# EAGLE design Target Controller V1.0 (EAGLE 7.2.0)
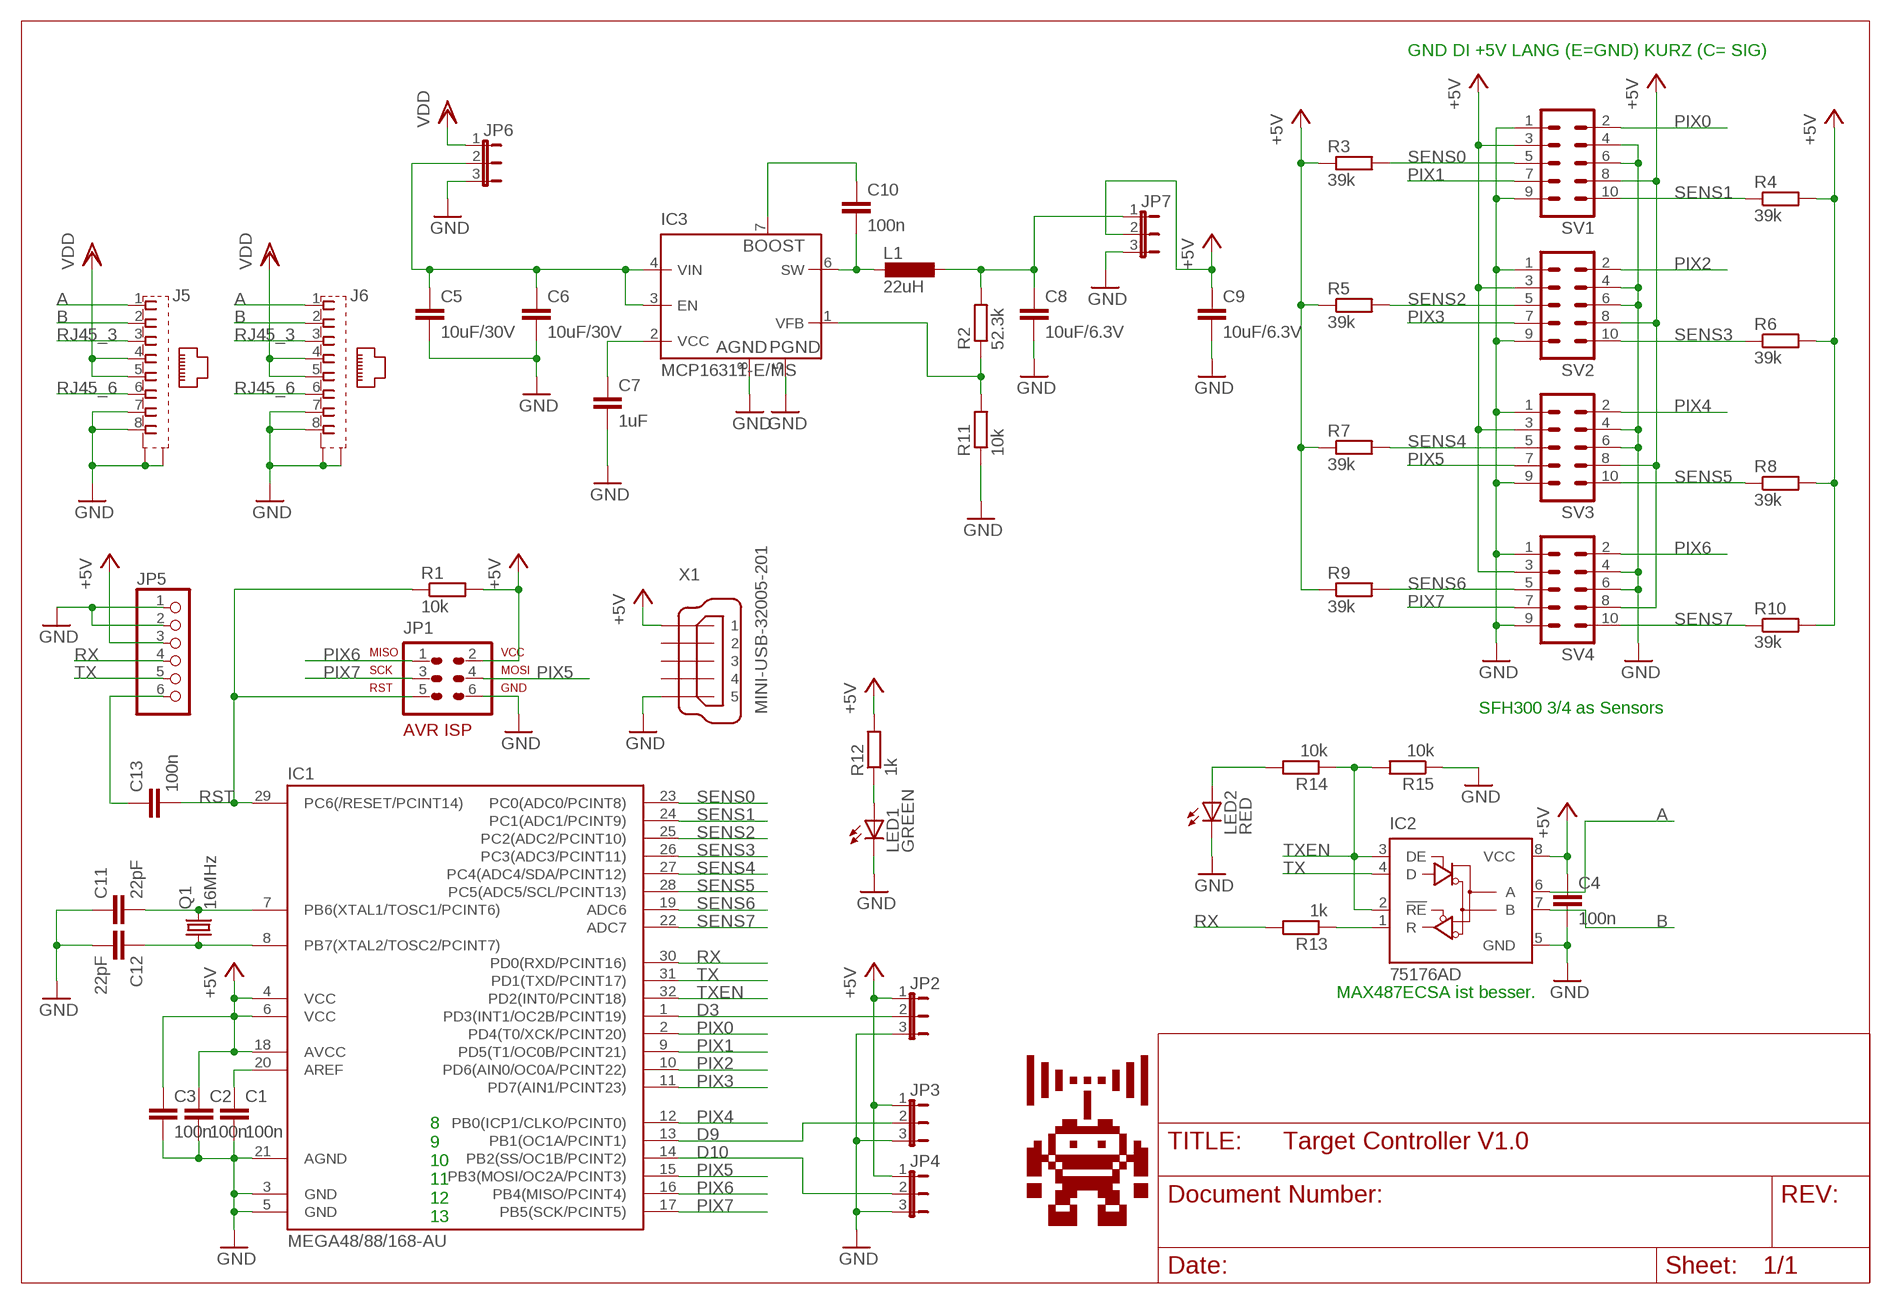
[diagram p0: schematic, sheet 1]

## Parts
C1  100n  C-EUC0805K  [C0805K]
C2  100n  C-EUC0805K  [C0805K]
C3  100n  C-EUC0805K  [C0805K]
C4  100n  C-EUC0805K  [C0805K]
C5  10uF/30V  C-EUC1206K  [C1206K]
C6  10uF/30V  C-EUC1206K  [C1206K]
C7  1uF  C-EUC0805K  [C0805K]
C8  10uF/6.3V  C-EUC0805K  [C0805K]
C9  10uF/6.3V  C-EUC0805K  [C0805K]
C10  100n  C-EUC0805K  [C0805K]
C11  22pF  C-EUC0603K  [C0603K]
C12  22pF  C-EUC0603K  [C0603K]
C13  100n  C-EUC0805K  [C0805K]
IC1  MEGA48/88/168-AU  [TQFP32-08]
IC2  75176AD  [D_R-PDSO-G8]
IC3  MCP16311-E/MS  MCP16311  [MSOP8]
J5  MEBP8-8G  [MEBP8-8G]
J6  MEBP8-8G  [MEBP8-8G]
JP1  AVR-ISP-6VERT  [AVR-ISP-6]
JP2  JP2E  [JP2]
JP3  JP2E  [JP2]
JP4  JP2E  [JP2]
JP5  PINHD-1X6  [1X06]
JP6  JP2E  [JP2]
JP7  JP2E  [JP2]
L1  22uH  L-PISM  [L-PISM22]
LED1  GREEN  LEDCHIPLED_0805  [CHIPLED_0805]
LED2  RED  LEDCHIPLED_0805  [CHIPLED_0805]
Q1  16MHz  CRYSTALHC49UP  [HC49UP]
R1  10k  R-EU_R0805  [R0805]
R2  52.3k  R-EU_R0805  [R0805]
R3  39k  R-EU_R0805  [R0805]
R4  39k  R-EU_R0805  [R0805]
R5  39k  R-EU_R0805  [R0805]
R6  39k  R-EU_R0805  [R0805]
R7  39k  R-EU_R0805  [R0805]
R8  39k  R-EU_R0805  [R0805]
R9  39k  R-EU_R0805  [R0805]
R10  39k  R-EU_R0805  [R0805]
R11  10k  R-EU_R0805  [R0805]
R12  1k  R-EU_R0805  [R0805]
R13  1k  R-EU_R0805  [R0805]
R14  10k  R-EU_R0805  [R0805]
R15  10k  R-EU_R0805  [R0805]
SV1  ML10L  [ML10L]
SV2  ML10L  [ML10L]
SV3  ML10L  [ML10L]
SV4  ML10L  [ML10L]
U$1  HACKFFM_LOGOLOGO_BSTOP  [LOGO_BSTOP]
X1  MINI-USB-32005-201  [32005-201]

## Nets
+5V: C2.1 C3.1 C4.1 C9.1 IC1.4(VCC) IC1.6(VCC) IC1.18(AVCC) IC2.8(VCC) JP1.2 JP2.1 JP3.1 JP4.1 JP5.3 JP7.2 R1.2 R3.1 R4.2 R5.1 R6.2 R7.1 R8.2 R9.1 R10.2 R12.2 SV1.3 SV1.8 SV2.3 SV2.8 SV3.3 SV3.8 SV4.3 SV4.8 X1.1
A: IC2.6(A) J5.1 J6.1
AREF: C1.1 IC1.20(AREF)
B: IC2.7(B) J5.2 J6.2
D3: IC1.1(PD3(INT1/OC2B/PCINT19)) JP2.2
D9: IC1.13(PB1(OC1A/PCINT1)) JP3.2
D10: IC1.14(PB2(SS/OC1B/PCINT2)) JP4.2
GND: C1.2 C2.2 C3.2 C4.2 C5.2 C6.2 C7.2 C8.2 C9.2 C11.1 C12.2 IC1.3(GND) IC1.5(GND) IC1.21(AGND) IC2.5(GND) IC3.5(PGND) IC3.8(AGND) J5.7 J5.8 J5.S1 J5.S2 J6.7 J6.8 J6.S1 J6.S2 JP1.6 JP2.3 JP3.3 JP4.3 JP5.1 JP5.2 JP6.3 JP7.3 LED1.C LED2.C R11.1 R15.1 SV1.1 SV1.4 SV1.6 SV1.9 SV2.1 SV2.4 SV2.6 SV2.9 SV3.1 SV3.4 SV3.6 SV3.9 SV4.1 SV4.4 SV4.6 SV4.9 X1.5
N$8: C10.1 IC3.7(BOOST)
N$9: C7.1 IC3.2(VCC)
N$11: C8.1 JP7.1 L1.2 R2.2
N$12: C12.1 IC1.8(PB7(XTAL2/TOSC2/PCINT7)) Q1.1
N$13: C11.2 IC1.7(PB6(XTAL1/TOSC1/PCINT6)) Q1.2
N$14: IC2.1(R) R13.1
N$15: LED1.A R12.1
N$16: C13.1 JP5.6
N$17: LED2.A R14.2
PIX0: IC1.2(PD4(T0/XCK/PCINT20)) SV1.2
PIX1: IC1.9(PD5(T1/OC0B/PCINT21)) SV1.7
PIX2: IC1.10(PD6(AIN0/OC0A/PCINT22)) SV2.2
PIX3: IC1.11(PD7(AIN1/PCINT23)) SV2.7
PIX4: IC1.12(PB0(ICP1/CLKO/PCINT0)) SV3.2
PIX5: IC1.15(PB3(MOSI/OC2A/PCINT3)) JP1.4 SV3.7
PIX6: IC1.16(PB4(MISO/PCINT4)) JP1.1 SV4.2
PIX7: IC1.17(PB5(SCK/PCINT5)) JP1.3 SV4.7
RJ45_3: J5.3 J6.3
RJ45_6: J5.6 J6.6
RST: C13.2 IC1.29(PC6(/RESET/PCINT14)) JP1.5 R1.1
RX: IC1.30(PD0(RXD/PCINT16)) JP5.4 R13.2
SENS0: IC1.23(PC0(ADC0/PCINT8)) R3.2 SV1.5
SENS1: IC1.24(PC1(ADC1/PCINT9)) R4.1 SV1.10
SENS2: IC1.25(PC2(ADC2/PCINT10)) R5.2 SV2.5
SENS3: IC1.26(PC3(ADC3/PCINT11)) R6.1 SV2.10
SENS4: IC1.27(PC4(ADC4/SDA/PCINT12)) R7.2 SV3.5
SENS5: IC1.28(PC5(ADC5/SCL/PCINT13)) R8.1 SV3.10
SENS6: IC1.19(ADC6) R9.2 SV4.5
SENS7: IC1.22(ADC7) R10.1 SV4.10
SW: C10.2 IC3.6(SW) L1.1
TX: IC1.31(PD1(TXD/PCINT17)) IC2.4(D) JP5.5
TXEN: IC1.32(PD2(INT0/PCINT18)) IC2.2(!RE) IC2.3(DE) R14.1 R15.2
VDD: J5.4 J5.5 J6.4 J6.5 JP6.1
VFB: IC3.1(VFB) R2.1 R11.2
VIN: C5.1 C6.1 IC3.3(EN) IC3.4(VIN) JP6.2
Unconnected: X1.2 X1.3 X1.4

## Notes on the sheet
- GND DI +5V LANG (E=GND) KURZ (C= SIG)
- SFH300 3/4 as Sensors
- MAX487ECSA ist besser.
- 8
  9
  10
  11
  12
  13

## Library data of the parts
C1-C13 = rcl:C-EU: CAPACITOR, European symbol
IC1 = avr-7:MEGA48/88/168
IC2 = 751xx:75176A: DIFFERENTIAL BUS TRANSCEIVER Source: http://focus.ti.com/lit/ds/symlink/sn75176a.pdf
IC3 = Lutz:MCP16311
J5 J6 = Lutz:MEBP8-8G
JP1 = avr-7:AVR-ISP-6: AVR ISP-6 Serial Programming Header
JP2-JP4 JP6 JP7 = jumper:JP2E: JUMPER
JP5 = pinhead:PINHD-1X6: PIN HEADER
L1 = Lutz:L-PISM
LED1 LED2 = led:LED: LED
Q1 = crystal:CRYSTAL: CRYSTAL; OC_FARNELL: unknown; OC_NEWARK: unknown
R1-R15 = rcl:R-EU_: RESISTOR, European symbol
SV1-SV4 = con-ml:ML10L: HARTING; OC_FARNELL: unknown; OC_NEWARK: unknown
U$1 = hackffm_logo:HACKFFM_LOGO
X1 = con-cypressindustries:MINI-USB-: MINI USB-B Conector Source: www.cypressindustries.com; OC_FARNELL: unknown; OC_NEWARK: unknown

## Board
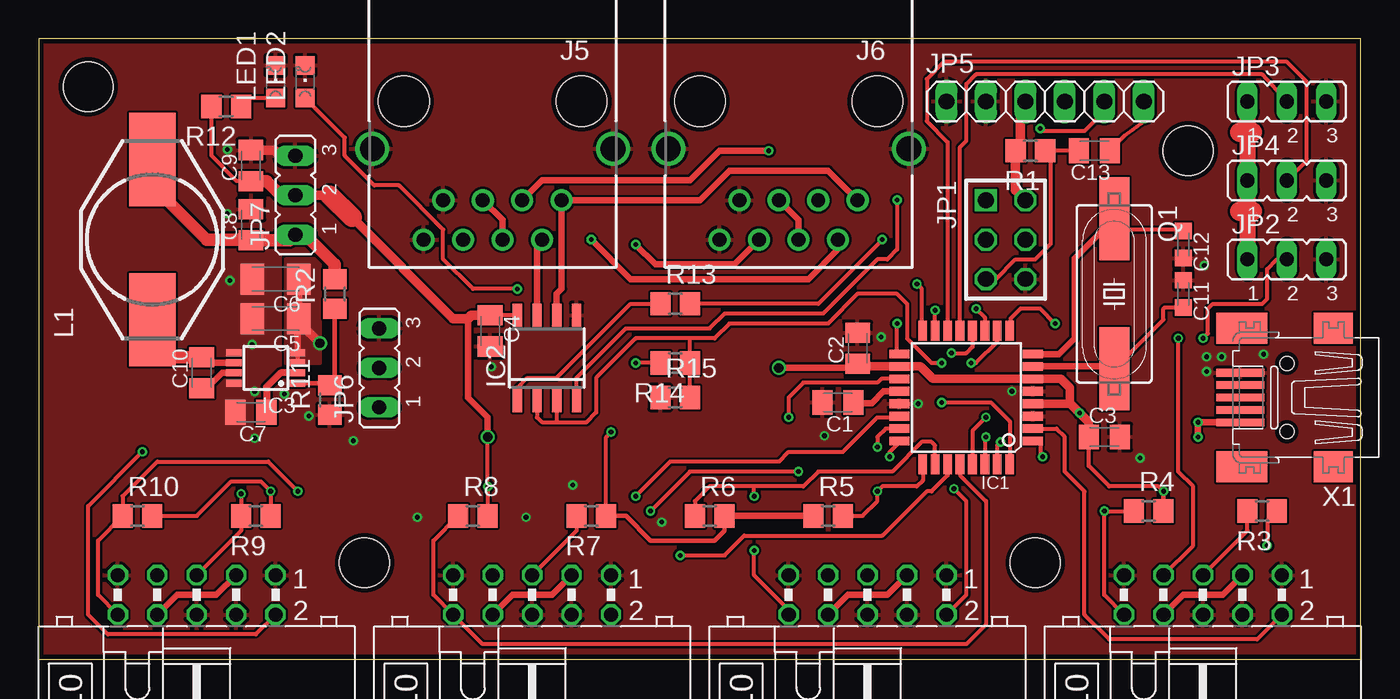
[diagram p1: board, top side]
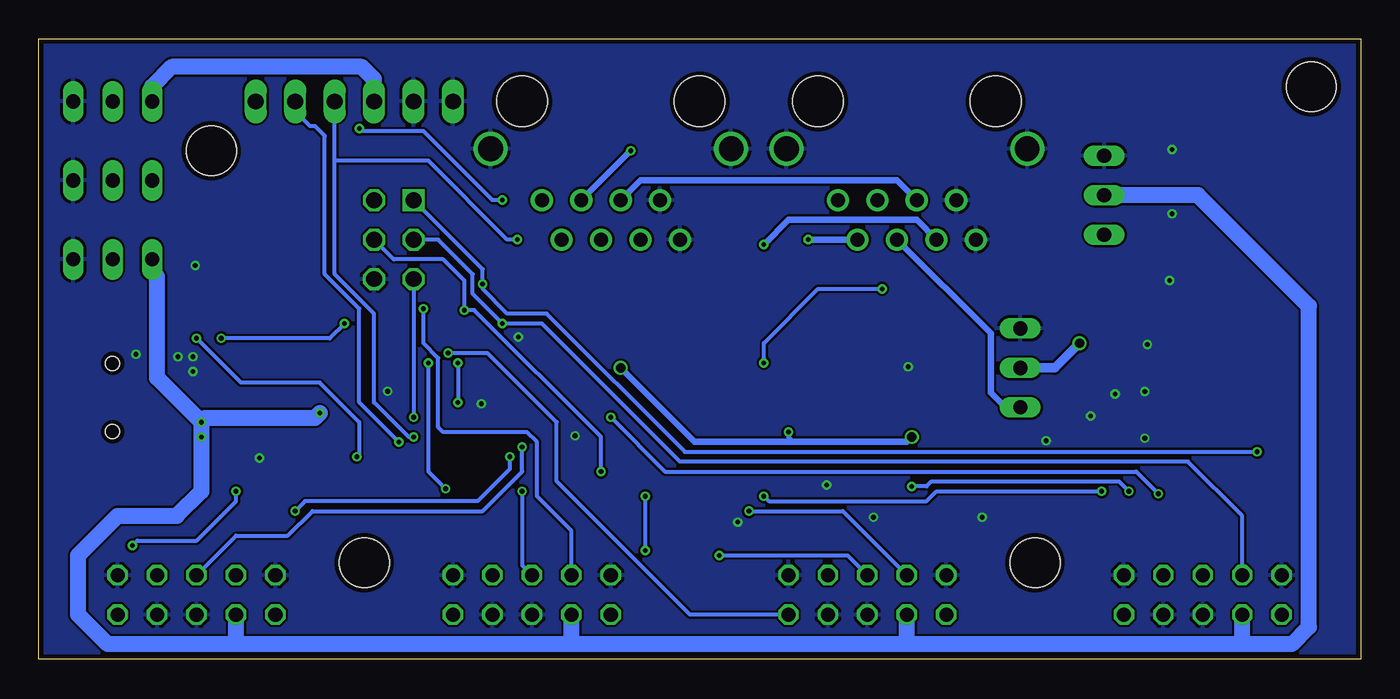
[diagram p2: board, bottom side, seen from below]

Size 85.08 x 39.91 mm. Coordinates in mm from the lower left corner, seen from the top.
Outline: 0,0 85.08,0 85.08,39.91 0,39.91 0,0
Copper layers (1*16): Top 0.035mm / dielectric 1.5mm / Bottom 0.035mm
Design rules "PCB-POOL Standard *": minimum track width 0.15mm, minimum drill 0.3mm, track to track 0.15mm, track to pad 0.15mm, pad to pad 0.15mm, via to via 0.15mm, smd to smd 0.15mm, copper to edge 0.3mm, drill to drill 0.2mm, minimum pad ring 0.2mm, minimum via ring 0.15mm, stop-mask expansion 0.075mm, vias tented up to drill 0.3mm, thermal gap 0.2mm
Holes 3.2 mm at 3.17,36.83 73.98,32.7 64.14,6.19 20.95,6.19

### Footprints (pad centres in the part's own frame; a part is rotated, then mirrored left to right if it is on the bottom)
C0805K = smd 1.3 x 1.6: 1 -1,0; 2 1,0
C1206K = smd 1.5 x 2: 1 -1.5,0; 2 1.5,0
C0603K = smd 1.05 x 1.08: 1 -0.875,0; 2 0.875,0
TQFP32-08 = smd 1.27 x 0.559: 1 -4.293,2.8; 2 -4.293,2; 3 -4.293,1.2; 4 -4.293,0.4; 5 -4.293,-0.4; 6 -4.293,-1.2; 7 -4.293,-2; 8 -4.293,-2.8; 17 4.293,-2.8; 18 4.293,-2; 19 4.293,-1.2; 20 4.293,-0.4; 21 4.293,0.4; 22 4.293,1.2; 23 4.293,2; 24 4.293,2.8 | smd 0.559 x 1.27: 9 -2.8,-4.293; 10 -2,-4.293; 11 -1.2,-4.293; 12 -0.4,-4.293; 13 0.4,-4.293; 14 1.2,-4.293; 15 2,-4.293; 16 2.8,-4.293; 25 2.8,4.293; 26 2,4.293; 27 1.2,4.293; 28 0.4,4.293; 29 -0.4,4.293; 30 -1.2,4.293; 31 -2,4.293; 32 -2.8,4.293
D_R-PDSO-G8 = smd 0.6 x 1.5: 1 -1.905,-2.75; 2 -0.635,-2.75; 3 0.635,-2.75; 4 1.905,-2.75; 5 1.905,2.75; 6 0.635,2.75; 7 -0.635,2.75; 8 -1.905,2.75
MSOP8 = smd 0.45 x 1: 1 -0.975,-2.05; 2 -0.325,-2.05; 3 0.325,-2.05; 4 0.975,-2.05; 5 0.975,2.05; 6 0.325,2.05; 7 -0.325,2.05; 8 -0.975,2.05
MEBP8-8G = drill 0.9 pad 1.422: 1 -4.445,-2.54; 2 -3.175,0; 3 -1.905,-2.54; 4 -0.635,0; 5 0.635,-2.54; 6 1.905,0; 7 3.175,-2.54; 8 4.445,0 | drill 1.6 pad 2.184: S1 -7.745,-5.84; S2 7.745,-5.84 | hole 3.25: 5.715,-8.89; -5.715,-8.89
AVR-ISP-6 = drill 1.016 square: 1 -2.54,-1.27 | drill 1.016 octagon: 2 -2.54,1.27; 3 0,-1.27; 4 0,1.27; 5 2.54,-1.27; 6 2.54,1.27
JP2 = drill 0.914 long: 1 -2.54,0; 2 0,0; 3 2.54,0
1X06 = drill 1.016 long: 1 -6.35,0; 2 -3.81,0; 3 -1.27,0; 4 1.27,0; 5 3.81,0; 6 6.35,0
L-PISM22 = smd 6 x 3: 1 -5.15,0; 2 5.15,0
CHIPLED_0805 = smd 1.2 x 1.2: A 0,-1.05; C 0,1.05
HC49UP = smd 5.334 x 1.93: 1 -4.826,0; 2 4.826,0
R0805 = smd 1.3 x 1.5: 1 -0.95,0; 2 0.95,0
ML10L = drill 0.914 octagon: 1 -5.08,-1.27; 2 -5.08,1.27; 3 -2.54,-1.27; 4 -2.54,1.27; 5 0,-1.27; 6 0,1.27; 7 2.54,-1.27; 8 2.54,1.27; 9 5.08,-1.27; 10 5.08,1.27
32005-201 = smd 3.1 x 0.5: 1 3,1.6; 2 3,0.8; 3 3,0; 4 3,-0.8; 5 3,-1.6 | smd 2.5 x 2: M1 -3,-4.45; M2 -3,4.45 | smd 3.3 x 2: M3 2.9,4.45; M4 2.9,-4.45 | hole 0.9: 0,2.2; 0,-2.2

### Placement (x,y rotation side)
C1  51.44,16.51 180 top
C2  52.7,20 90 top
C3  68.58,14.29 0 top
C4  29.05,21.11 270 top
C5  15.24,21.91 180 top
C6  15.24,24.45 180 top
C7  13.65,15.88 180 top
C8  13.65,27.94 90 top
C9  13.65,31.75 90 top
C10  10.48,18.41 90 top
C11  73.66,23.5 270 top
C12  73.66,26.67 270 top
C13  67.94,32.7 180 top
IC1  59.69,16.83 180 top
IC2  32.7,19.37 0 top
IC3  14.61,18.73 90 top
J5  29.21,26.99 180 top
J6  48.26,26.99 180 top
JP1  62.23,26.99 270 top
JP2  80.33,25.72 0 top
JP3  80.33,35.88 0 top
JP4  80.33,30.8 0 top
JP5  64.77,35.88 0 top
JP6  21.91,18.73 90 top
JP7  16.51,29.84 90 top
L1  7.3,26.99 90 top
LED1  15.24,37.15 0 top
LED2  17.14,37.15 0 top
Q1  69.22,23.5 270 top
R1  63.82,32.7 180 top
R2  19.05,23.5 90 top
R3  78.74,9.53 180 top
R4  71.44,9.53 0 top
R5  50.8,9.21 0 top
R6  43.18,9.21 0 top
R7  35.56,9.21 180 top
R8  27.94,9.21 0 top
R9  13.97,9.21 180 top
R10  6.35,9.21 0 top
R11  18.73,16.67 90 top
R12  12.06,35.56 180 top
R13  40.96,22.86 0 top
R14  40.96,19.05 180 top
R15  40.96,16.83 0 top
SV1  74.93,4.13 180 top
SV2  53.34,4.13 180 top
SV3  31.75,4.13 180 top
SV4  10.16,4.13 180 top
U$1  8.73,19.68 270 top
X1  80.33,16.83 180 top

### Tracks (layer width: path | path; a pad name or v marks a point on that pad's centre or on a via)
+5V  (via drill 0.3, 0.6)
  Top 0.254: 78.11,28.81 77.79,29.13 77.79,31.75 | 78.11,33.89 77.79,34.21 JP3.1 | v72.39,10.79 R4.2 v72.39,10.79 | v72.39,10.79 72.07,11.11 68.9,11.11 67.58,12.43 C3.1 | R3.1 79.06,8.89 v79.06,7.3 | IC2.8 C4.1 | C9.1 12.75,30.75 11.11,32.38 R12.2 | R10.2 10.16,9.21 12.38,11.43 14.29,11.43 v14.92,10.79 R9.1 | v28.89,14.29 v28.89,11.11 R8.2 | R7.1 36.51,14.29 v36.83,14.61
  Top 0.305: R7.1 37.78,9.21 39.37,7.62 43.5,7.62 44.13,8.26 R6.2
  Top 0.406: SV4.8 8.89,4.13 11.43,4.13 SV4.3 | SV3.8 30.48,4.13 33.02,4.13 SV3.3 | SV2.8 52.07,4.13 54.61,4.13 SV2.3 | SV1.8 73.66,4.13 76.2,4.13 SV1.3 | X1.1 77.31,15.24 v74.61,15.24 v74.61,14.29 | 49.53,8.89 R5.1 R6.2 | R10.2 | R9.1 | R8.2 | C2.1 52.44,19 | 52.44,18.73 v47.62,18.73 | 27.62,21.91 27.62,16.83 28.89,15.56 v28.89,14.29
  Top 0.559: C2.1 52.53,18.83 IC1.18 56.74,18.83 57.54,18.03 IC1.6 65.79,18.03 66.36,17.46 66.36,16.46 v66.99,15.83 | IC1.4 66.39,16.43 v66.99,15.83 | C3.1 67.58,15.24 v66.99,15.83
  Top 0.61: JP7.2 18.73,29.84 | JP5.3 63.18,35.56 63.18,33.02 R1.2 62.87,30.16 JP1.2 | 20.16,28.42 26.67,21.91 27.62,21.91 27.83,22.12 C4.1 | C2.1 52.44,18.73
  Top 0.813: C9.1 14.65,30.75 15.56,29.84 JP7.2
  Top 1.016: JP2.1 JP4.1 77.79,31.75 JP3.1
  Top 1.27: 18.73,29.84 20.16,28.42 | 77.31,33.89 78.11,33.89 | 77.31,28.81 78.11,28.81
  Bottom 0.254: v79.06,7.3 78.74,7.62 74.93,7.62 72.39,10.16 v72.39,10.79 | v14.92,10.79 15.56,11.43 27.62,11.43 27.94,11.11 v28.89,11.11 | v36.83,14.61 36.83,14.29 36.51,13.97
  Bottom 0.406: v28.89,14.29 29.21,13.97 36.51,13.97 42.86,13.97 v47.62,18.73
  Bottom 1.016: 7.62,0.95 4.45,0.95 3.33,2.06 3.33,22.7 10.48,29.84 JP7.2 | 7.62,0.95 29.21,0.95 | 29.21,0.95 50.8,0.95 | 50.8,0.95 72.39,0.95 | 72.39,0.95 80.64,0.95 82.55,2.86 82.55,6.67 80.01,9.21 76.2,9.21 74.61,10.79 v74.61,15.24 | 72.39,0.95 SV1.8 | 50.8,0.95 SV2.8 | 29.21,0.95 SV3.8 | 7.62,0.95 SV4.8 | v74.61,15.24 77.47,18.1 77.47,24.61 77.79,24.92 JP2.1 | v74.61,15.24 74.34,15.51 67.31,15.51 v66.99,15.83 | JP5.3 63.5,37.31 64.29,38.1 76.52,38.1 77.79,36.83 JP3.1
A
  Top 0.406: IC2.6 33.34,23.5 33.66,23.81 J5.1 42.55,29.53 44.45,31.43 50.8,31.43 J6.1
AREF
  Top 0.406: IC1.20 54.38,17.23 53.61,16.46 52.48,16.46 C1.1
B  (via drill 0.3)
  Top 0.406: J5.2 32.07,26.67 IC2.7 | v35.56,26.99 38.1,24.45 49.53,24.45 51.44,26.35 J6.2
  Bottom 0.406: J5.2 v35.56,26.99
D3  (via drill 0.3)
  Top 0.254: IC1.1 64.45,14.03 64.45,13.18 v64.61,13.02 | v74.93,20.64 75.25,20.95 75.25,22.54 75.56,22.86 78.74,22.86 79.06,23.18 79.06,25.08 79.69,25.72 JP2.2
  Bottom 0.254: v64.61,13.02 64.45,13.18 64.45,15.24 66.99,17.78 72.07,17.78 v74.93,20.64
D9
  Top 0.254: JP3.2 78.74,37.62 60.33,37.62 59.69,36.99 59.69,33.34 59.29,32.94 IC1.13
D10
  Top 0.254: JP4.2 81.6,32.07 81.6,37.15 80.33,38.42 58.26,38.42 57.15,37.31 57.15,34.61 58.49,33.27 IC1.14
GND  (via drill 0.3)
  Top 0.406: IC3.8 12.34,17.76
  Top 0.61: C9.2 15.19,32.75 15.56,32.38 JP7.3
  other vias: 56.6,16.43 62.63,17.23 13.73,20.24 13.89,17.22 17.39,15.63 13.89,14.21 15.8,17.06 12.15,32.78 12.15,28.65 12.31,24.36 31.36,9.12 24.37,9.12 40.09,8.81 34.37,11.19 20.24,14.05 29.13,18.81 78.82,19.61 76.12,19.45 70.89,12.94 54.22,20.72 75.01,25.32 75.17,19.45 75.17,18.5 50.56,14.36
  pour Bottom: 0,0 0,40.64 85.09,40.64 85.09,0
  pour Top (rank 2): 0,0 0,40.64 85.09,40.64 85.09,0
  pour Top (no thermals): 11.75,25.72 14.92,25.72 14.92,14.61 11.43,14.61 11.43,25.72
N$8
  Top 0.406: IC3.7 11.79,18.41 10.79,17.41 C10.1
N$9
  Top 0.457: IC3.2 15.55,18.41 14.65,17.51 C7.1
N$11
  Top 0.813: 7.62,31.43 L1.2 6.99,30.8 10.79,26.99 13.61,26.99 C8.1 16.14,26.94 JP7.1 17.14,27.3 19.05,25.4 R2.2
N$12
  Top 0.254: C12.1 73.58,27.62 69.22,27.62
  Top 0.406: 69.22,26.04 69.22,27.62 Q1.1 | 69.22,27.86 Q1.1 | IC1.8 65.67,19.63 66.67,20.64 66.67,25.78 Q1.1 | 69.39,28.18 Q1.1
N$13
  Top 0.254: Q1.2 72.39,21.84 72.39,22.54 72.47,22.62 C11.2
  Top 0.406: IC1.7 69.22,18.83 Q1.2 69.22,21.03
N$14
  Top 0.254: R13.1 38.1,22.86 33.34,18.1 31.43,18.1 30.8,17.46 IC2.1
N$15
  Top 0.254: LED1.A 13.55,36.1 R12.1
N$16
  Top 0.254: C13.1 69.9,33.7 71.12,34.61 JP5.6
N$17  (via drill 0.3)
  Top 0.254: R14.2 v38.42,19.05 | v30.8,23.81 27.94,23.81 26.04,25.72 26.04,27.62 23.18,30.48 21.59,30.48 19.68,32.38 19.68,33.56 LED2.A
  Bottom 0.254: v38.42,19.05 38.42,20.32 34.92,23.81 v30.8,23.81
PIX0
  Top 0.254: IC1.2 65.5,14.83 66.04,14.29 66.04,12.06 67.31,10.79 67.31,2.86 68.9,1.27 78.42,1.27 SV1.2
PIX1  (via drill 0.3)
  Top 0.254: 62.49,21.59 IC1.9 62.49,21.53 62.55,21.59 62.55,21.91 63.18,22.54 64.45,22.54 v65.41,21.59 | v73.34,20.64 73.34,12.06 74.3,11.11 74.3,7.3 SV1.7
  Bottom 0.254: v65.41,21.59 66.36,20.64 v73.34,20.64
PIX2  (via drill 0.3)
  Top 0.254: IC1.10 61.69,20.41 60.33,19.05 v60.01,19.05 | SV2.2 59.69,4.13 59.69,10.16 v58.9,10.95
  Bottom 0.254: v58.9,10.95 60.01,12.06 v60.01,19.05
PIX3  (via drill 0.3)
  Top 0.254: v60.33,22.54 60.89,21.98 IC1.11
  Bottom 0.254: SV2.7 50.8,8.26 53.02,10.48 53.02,13.97 53.66,14.61 59.05,14.61 59.37,14.92 59.37,19.37 60.33,20.32 v60.33,22.54
PIX4  (via drill 0.3)
  Top 0.254: IC1.12 60.09,20.09 59.69,19.68 v58.74,19.68
  Bottom 0.254: SV3.2 43.18,2.86 51.75,11.43 51.75,15.24 56.2,19.68 v58.74,19.68
PIX5  (via drill 0.3)
  Top 0.254: IC1.15 v57.69,22.45 | v48.9,12.06 41.91,12.06 v39.37,9.53
  Bottom 0.254: JP1.4 62.23,25.72 59.05,25.72 57.69,24.35 v57.69,22.45 57.05,22.45 48.9,14.29 v48.9,12.06 | v39.37,9.53 33.34,9.53 SV3.7
PIX6  (via drill 0.3)
  Top 0.254: SV4.2 13.97,1.59 4.45,1.59 3.17,2.86 3.17,9.84 v6.67,13.34 | 56.83,21.18 56.83,23.81 v56.52,24.13
  Top 0.406: 56.83,21.18 IC1.16
  Bottom 0.254: v6.67,13.34 43.5,13.34 52.39,22.23 54.93,22.23 56.52,23.81 v56.52,24.13 56.52,25.08 JP1.1
PIX7  (via drill 0.3)
  Top 0.254: IC1.17 55.24,19.63 v55.24,21.59
  Bottom 0.254: JP1.3 59.37,26.99 57.15,24.77 57.15,23.5 v55.24,21.59 52.7,21.59 43.81,12.7 11.11,12.7 7.62,9.21 SV4.7
RJ45_3  (via drill 0.3)
  Top 0.406: J5.3 32.38,30.8 41.91,30.8 43.81,32.7 v46.99,32.7
  Bottom 0.406: J6.3 v46.99,32.7
RJ45_6  (via drill 0.3)
  Top 0.406: v38.42,26.67 39.69,25.4 44.77,25.4 J6.6
  Bottom 0.406: J5.6 28.57,28.26 36.83,28.26 v38.42,26.67
RST  (via drill 0.3)
  Top 0.254: IC1.29 60.09,14.69 v60.96,15.56 | JP1.5 61.59,24.45 62.87,25.72 64.14,25.72 65.13,26.71 65.13,32.59 R1.1 C13.2
  Bottom 0.254: JP1.5 v60.96,15.56
RX  (via drill 0.3)
  Top 0.254: v60.96,14.29 60.89,14.22 IC1.30 | v54.29,26.99 50.16,22.86 R13.2
  Bottom 0.254: 66.04,32.07 66.04,24.77 63.5,22.23 63.5,16.51 61.28,14.29 v60.96,14.29 | 66.04,32.07 JP5.4 | v54.29,26.99 54.93,26.99 60.01,32.07 66.04,32.07
SENS0  (via drill 0.3)
  Top 0.254: SV1.5 77.79,8.26 R3.2 | IC1.23 54.52,14.83 53.98,14.29 v53.98,13.65
  Bottom 0.254: SV1.5 72.39,7.94 69.06,7.94 67.47,9.53 56.52,9.53 53.98,12.06 v53.98,13.65
SENS1  (via drill 0.3)
  Top 0.254: SV1.10 68.58,4.13 v68.58,9.53 R4.1 | IC1.24 55.46,14.03 54.77,13.34 v54.77,13.02
  Bottom 0.254: v68.58,9.53 67.94,10.16 56.83,10.16 54.77,12.22 v54.77,13.02
SENS2  (via drill 0.3)
  Top 0.254: IC1.25 56.89,11.49 56.52,11.11 54.29,11.11 v53.98,10.79 53.98,10.16 53.02,9.21 R5.2
  Bottom 0.254: v53.98,10.79 53.98,6.03 SV2.5
SENS3  (via drill 0.3)
  Top 0.254: 42.23,8.89 R6.1 42.23,10.16 43.18,11.11 46.04,11.11 | IC1.26 57.69,13.75 57.47,13.97 56.83,13.97 54.93,12.06 50.16,12.06 49.21,11.11 46.04,11.11 | SV2.10 48.26,3.17 46.04,5.4 v46.04,6.99 | v46.04,10.48 46.04,11.11
  Bottom 0.254: v46.04,6.99 v46.04,10.48
SENS4  (via drill 0.3)
  Top 0.254: R7.2 34.61,8.26 SV3.5 | v41.27,6.67 44.13,6.67 45.4,7.94 54.29,7.94 57.15,10.79 57.47,10.79 58.49,11.82 IC1.27
  Bottom 0.254: v41.27,6.67 33.02,6.67 32.7,6.35 SV3.5
SENS5
  Top 0.254: R8.1 25.4,7.62 25.4,4.13 SV3.10 28.57,0.95 59.69,0.95 60.96,2.22 60.96,10.16 59.29,11.83 IC1.28
SENS6  (via drill 0.3)
  Top 0.254: IC1.19 54.22,18.03 53.98,17.78 49.21,17.78 48.26,16.83 v48.26,15.56 | v13.02,10.64 R9.2 13.02,8.26 SV4.5
  Bottom 0.254: v48.26,15.56 44.77,12.06 14.45,12.06 v13.02,10.64
SENS7  (via drill 0.3)
  Top 0.254: SV4.10 3.81,4.13 3.81,7.62 R10.1 5.4,10.48 7.62,12.7 14.76,12.7 v16.67,10.79 | IC1.22 55.33,15.56 53.98,15.56 51.75,13.34 48.26,13.34 47.62,12.7 40.64,12.7 v38.42,10.48
  Bottom 0.254: v38.42,10.48 38.1,10.16 27.94,10.16 27.3,10.79 v16.67,10.79
SW
  Top 0.406: IC3.6 10.79,19.06 10.48,19.37 10.84,19.37 C10.2
  Top 0.813: C10.2 7.57,19.41 7.62,20.64 L1.1
TX  (via drill 0.3)
  Top 0.254: IC1.31 61.69,13.75 v61.91,13.97 | JP5.5 68.58,35.24 67.31,33.97 64.61,33.97 v64.45,34.13 | v55.24,29.53 55.24,26.35 54.61,25.72 53.98,25.72 50.48,22.23 44.13,22.23 43.18,21.27 37.78,21.27 34.61,18.1 IC2.4
  Bottom 0.254: v61.91,13.97 64.45,16.51 64.45,22.54 66.67,24.77 66.67,33.66 67.31,34.29 67.63,34.29 68.58,35.24 JP5.5 | v55.24,29.53 55.88,29.53 60.33,33.97 64.29,33.97 v64.45,34.13
TXEN  (via drill 0.3)
  Top 0.254: v58.1,16.51 61.28,16.51 62.49,15.3 IC1.32 | v58.1,19.05 57.47,19.05 55.88,20.64 55.88,22.86 55.24,23.5 52.7,23.5 50.8,21.59 44.45,21.59 43.5,20.64 41.91,20.64 | IC2.2 32.07,15.56 32.38,15.24 33.34,15.24 | 33.34,15.24 35.24,15.24 35.88,15.88 35.88,18.1 38.42,20.64 41.91,20.64 | IC2.3 33.34,15.24 | 41.91,20.64 R14.1 R15.2
  Bottom 0.254: v58.1,19.05 v58.1,16.51
VDD
  Top 0.406: J6.5 48.9,28.26 J6.4 | J5.5 29.84,28.26 J5.4
  Bottom 0.406: J6.5 46.35,30.8 29.84,30.8 J5.5 | JP6.1 22.86,16.19 23.81,17.14 23.81,20.95 J5.4
VFB
  Top 0.305: IC3.1 18.39,17.76 18.41,17.78 | 18.41,17.78 R11.2 | R2.1 19.05,17.78 18.41,17.78
VIN  (via drill 0.6)
  Top 0.305: IC3.4 IC3.3 16.66,21.1 16.83,21.59
  Top 0.406: IC3.4 16.66,21.1 16.66,21.82 C5.1 C6.1
  Top 0.61: 16.83,21.59 v18.1,20.32
  Bottom 0.61: v18.1,20.32 19.68,18.73 JP6.2
  pour Top (no thermals): 15.88,19.05 18.1,19.05 18.1,25.72 15.88,25.72

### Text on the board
tStop: PWR | TX | DTR | 5V | D9 | GND | GND | VCC | 5V | D10 | GND | 5V-STEP | 5V | D3 | GND | GND | VIN | Space'n'Lasers Target Controller | VRJ45 | 4 | 3 | 2 | 1
bStop: V1.0 by LL | Space'n'Lasers | Target Controller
